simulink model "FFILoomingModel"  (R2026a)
settings: Solver=ode1  StopTime=T_max  FixedStep=0.00001
libraries: LoomingNeuronLibrary x10

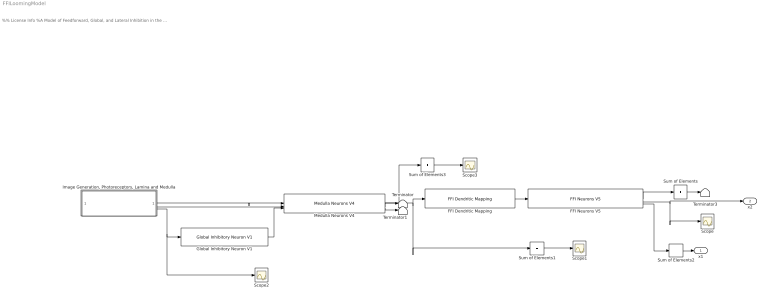
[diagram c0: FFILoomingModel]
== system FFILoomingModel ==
  note: %% License Info %A Model of Feedforward, Global, and Lateral Inhibition in the Locust Visual System. %This model examines the architecture and function of inhibitory mechanisms in the %visual system of locusts, namely those involved in the processing of inputs to a %key looming-sensitive neuron, the lobula giant movement detector (LGMD). %Copyright (c) 2026, Erik Olson, Travis Wiens, and Jack Gray %CITATION: %When using the model code for scientific publications, cite the following work: %Olson EGN, Wiens TK, Gray JR. A model of feedforward, global, and lateral inhibition %in the locust visual system predicts responses to looming stimuli. Biol Cybern. 2021 %Jun;115(3):245-265. doi: 10.1007/s00422-021-00876-8. Epub 2021 May 16. PMID: 33997912. %This program is free software: you can redistribute it and/or modify %it under the terms of the GNU General Public License as published by %the Free Software Foundation, either version 3 of the License, or %(at your option) any later version. %This program is distributed in the hope that it will be useful, %but WITHOUT ANY WARRANTY; without even the implied warranty of %MERCHANTABILITY or FITNESS FOR A PARTICULAR PURPOSE. See the %GNU General Public License for more details. %You should have received a copy of the GNU General Public License %along with this program. If not, see <https://www.gnu.org/licenses/>. %Contact: erik.olson@usask.ca
  FFI Dendritic Mapping : LoomingNeuronLibrary/FFI Dendritic Mapping  r_f=r_field  r_s=r_spacing  pop_FFI=pop_f
  FFI Neurons V5 : LoomingNeuronLibrary/FFI Neurons V5  K_in=K_E_f  g_m=g_L_f  c_m=c  E_rev=E_E  E_rest=E_L  V_t=V_t  Delta_t=Delta_t_f  V_fire=V_fire  tau=tau_alpha_f  g_FFI_adap=Delta_g_A_f  tau_FFI_adap=tau_A_f  E_adap=E_A  g_noise=g_N_f  noise_T=T_noise  pop=pop_f
  Global Inhibitory Neuron V1 : LoomingNeuronLibrary/Global Inhibitory Neuron V1  K_in=K_GI
  "Image Generation, Photoreceptors, Lamina and Medulla" : Subsystem  TreatAsAtomicUnit=on  SystemSampleTime=0.0004
  Medulla Neurons V4 : LoomingNeuronLibrary/Medulla Neurons V4  K_in_ex=K_E_m  K_in_lateral=K_lat_m  K_in_global=K_gl_m  g_m=g_L_m  c_m=c  E_rev_ex=E_E  E_rev_inh=E_I  E_rest=E_L  V_t=V_t  Delta_t=Delta_t_m  V_fire=V_fire  tau=tau_alpha_m  g_med_adap_inc=Delta_g_A_m  tau_med_adap=tau_A_m  E_rev_adap=E_A  g_noise=g_N_m  noise_T=T_noise  radius=radius
  Scope{,1..3} (4 alike) : Scope
  Sum of Elements{,1..3} (4 alike) : Sum  Inputs=+
  Terminator : Terminator
  Terminator1 : Terminator
  Terminator3 : Terminator
  x1 : Outport  VectorParamsAs1DForOutWhenUnconnected=off
  x2 : Outport  Port=2  VectorParamsAs1DForOutWhenUnconnected=off
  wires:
  "Image Generation, Photoreceptors, Lamina and Medulla"/2(Lateral Inhibition) -> Medulla Neurons V4/2
  Medulla Neurons V4/1 -> Sum of Elements3/1, Sum of Elements1/1, FFI Dendritic Mapping/1
  Medulla Neurons V4/2 -> Terminator/1
  FFI Dendritic Mapping/1 -> FFI Neurons V5/1
  FFI Neurons V5/2 -> Scope/1, x2/1
  Sum of Elements/1 -> Terminator3/1
  Sum of Elements1/1 -> Scope1/1
  Medulla Neurons V4/3 -> Terminator1/1
  FFI Neurons V5/3 -> Sum of Elements2/1
  Sum of Elements2/1 -> x1/1
  FFI Neurons V5/1 -> Sum of Elements/1
  Global Inhibitory Neuron V1/1 -> Medulla Neurons V4/3
  "Image Generation, Photoreceptors, Lamina and Medulla"/1(Excitation) -> Medulla Neurons V4/1
  "Image Generation, Photoreceptors, Lamina and Medulla"/3(Global Inhibition) -> Global Inhibitory Neuron V1/1, Scope2/1
  Sum of Elements3/1 -> Scope3/1

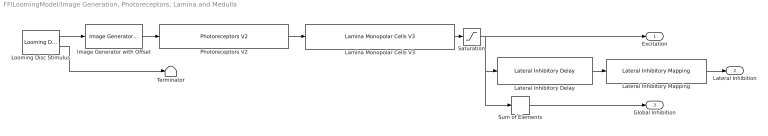
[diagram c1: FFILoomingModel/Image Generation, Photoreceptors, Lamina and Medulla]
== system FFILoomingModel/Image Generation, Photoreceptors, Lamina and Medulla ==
  Image Generator with Offset : LoomingNeuronLibrary/Image Generator with Offset  radius=radius  theta_max=theta_max  h_offset=h_offset  v_offset=v_offset
  Lamina Monopolar Cells V3 : LoomingNeuronLibrary/Lamina Monopolar Cells V3  K_LMC=K_LMC  gamma_1=b
  Lateral Inhibitory Delay : LoomingNeuronLibrary/Lateral Inhibitory Delay  tau=tau_lat
  Lateral Inhibitory Mapping : LoomingNeuronLibrary/Lateral Inhibitory Mapping  stencil=inhibitory_kernel
  Looming Disc Stimulus : LoomingNeuronLibrary/Looming Disc Stimulus  l=l  v=v  d_0=d
  Photoreceptors V2 : LoomingNeuronLibrary/Photoreceptors V2  K_photoD=K_photoD  K_photoP=K_photoP  alpha_1=a_1  alpha_2=a_2
  Saturation : Saturate  UpperLimit=inf  LowerLimit=0
  Sum of Elements : Sum  Inputs=+
  Terminator : Terminator
  Excitation : Outport  VectorParamsAs1DForOutWhenUnconnected=off
  Lateral Inhibition : Outport  Port=2  VectorParamsAs1DForOutWhenUnconnected=off
  Global Inhibition : Outport  Port=3  VectorParamsAs1DForOutWhenUnconnected=off
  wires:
  Image Generator with Offset/1 -> Photoreceptors V2/1
  Photoreceptors V2/1 -> Lamina Monopolar Cells V3/1
  Looming Disc Stimulus/2 -> Terminator/1
  Looming Disc Stimulus/1 -> Image Generator with Offset/1
  Lamina Monopolar Cells V3/1 -> Saturation/1
  Lateral Inhibitory Mapping/1 -> Lateral Inhibition/1
  Sum of Elements/1 -> Global Inhibition/1
  Lateral Inhibitory Delay/1 -> Lateral Inhibitory Mapping/1
  Saturation/1 -> Excitation/1, Sum of Elements/1, Lateral Inhibitory Delay/1
